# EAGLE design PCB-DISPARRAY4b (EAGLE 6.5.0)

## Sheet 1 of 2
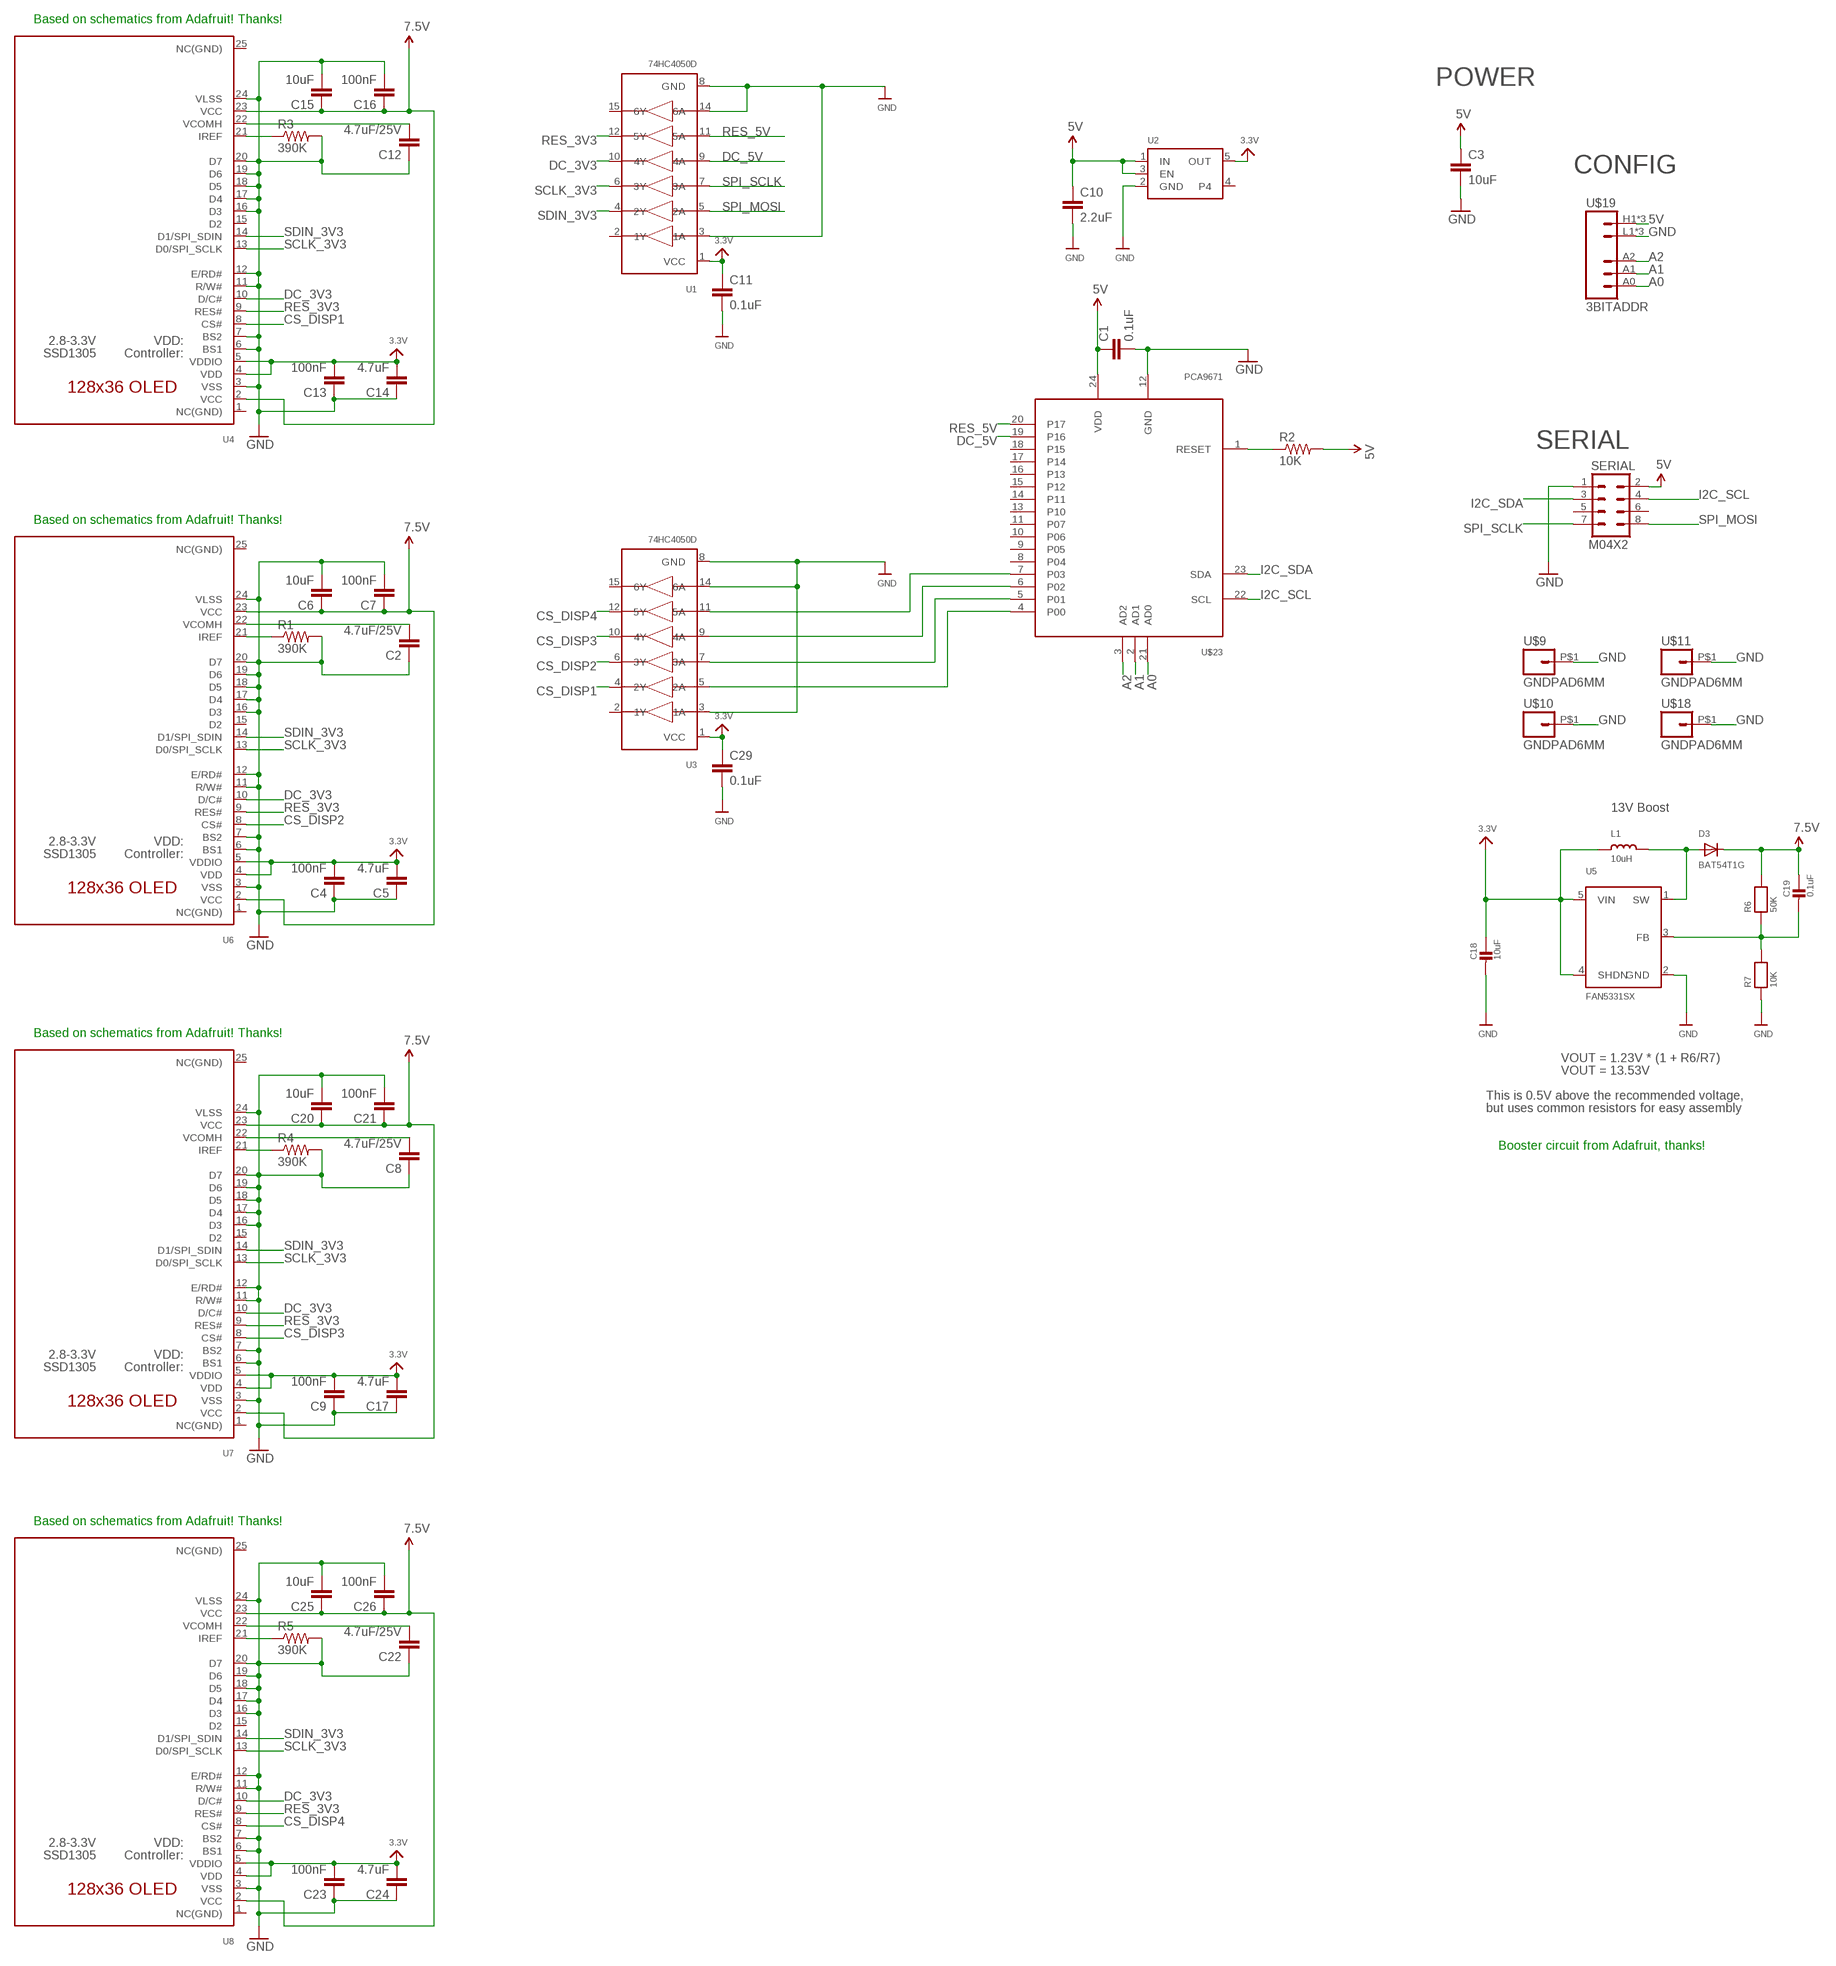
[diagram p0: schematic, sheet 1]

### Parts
C1  0.1uF  CAP0603-CAP  [0603-CAP]
C2  4.7uF/25V  CAP0805  [0805]
C3  10uF  CAP0805  [0805]
C4  100nF  CAP0603-CAP  [0603-CAP]
C5  4.7uF  CAP0603-CAP  [0603-CAP]
C6  10uF  CAP0603-CAP  [0603-CAP]
C7  100nF  CAP0603-CAP  [0603-CAP]
C8  4.7uF/25V  CAP0805  [0805]
C9  100nF  CAP0603-CAP  [0603-CAP]
C10  2.2uF  CAP0603-CAP  [0603-CAP]
C11  0.1uF  CAP0603-CAP  [0603-CAP]
C12  4.7uF/25V  CAP0805  [0805]
C13  100nF  CAP0603-CAP  [0603-CAP]
C14  4.7uF  CAP0603-CAP  [0603-CAP]
C15  10uF  CAP0603-CAP  [0603-CAP]
C16  100nF  CAP0603-CAP  [0603-CAP]
C17  4.7uF  CAP0603-CAP  [0603-CAP]
C18  10uF  CAP_CERAMIC0805  [0805]
C19  0.1uF  CAP_CERAMIC0805  [0805]
C20  10uF  CAP0603-CAP  [0603-CAP]
C21  100nF  CAP0603-CAP  [0603-CAP]
C22  4.7uF/25V  CAP0805  [0805]
C23  100nF  CAP0603-CAP  [0603-CAP]
C24  4.7uF  CAP0603-CAP  [0603-CAP]
C25  10uF  CAP0603-CAP  [0603-CAP]
C26  100nF  CAP0603-CAP  [0603-CAP]
C29  0.1uF  CAP0603-CAP  [0603-CAP]
D3  BAT54T1G  DIODESOD-123  [SOD-123]
L1  10uH  INDUCTOR  [INDUCTOR_1007]
R1  390K  RESISTOR0603-RES  [0603-RES]
R2  10K  RESISTOR0603-RES  [0603-RES]
R3  390K  RESISTOR0603-RES  [0603-RES]
R4  390K  RESISTOR0603-RES  [0603-RES]
R5  390K  RESISTOR0603-RES  [0603-RES]
R6  50K  RESISTOR0805  [0805]
R7  10K  RESISTOR0805  [0805]
SERIAL  M04X2  [2X4]
U1  74HC4050D  [SOIC16]
U2  VREG_SOT23-5  [SOT23-5]
U3  74HC4050D  [SOIC16]
U4  ER-OLED011-1  [ER-OLED011-1_WRAPAROUND]
U5  FAN5331SX  FAN5331  [SOT23-5@1]
U6  ER-OLED011-1  [ER-OLED011-1_WRAPAROUND]
U7  ER-OLED011-1  [ER-OLED011-1_WRAPAROUND]
U8  ER-OLED011-1  [ER-OLED011-1_WRAPAROUND]
U$9  GNDPAD6MM  [3.2MMPAD6MM]
U$10  GNDPAD6MM  [3.2MMPAD6MM]
U$11  GNDPAD6MM  [3.2MMPAD6MM]
U$18  GNDPAD6MM  [3.2MMPAD6MM]
U$19  3BITADDR  [3BITADDR]
U$23  PCA9671  [TSSOP24]

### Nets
3.3V: C4.2 C5.2 C9.2 C11.1 C13.2 C14.2 C17.2 C18.1 C23.2 C24.2 C29.1 L1.P$1 U1.1(VCC) U2.5(OUT) U3.1(VCC) U4.4(VDD) U4.5(VDDIO) U5.4(SHDN) U5.5(VIN) U6.4(VDD) U6.5(VDDIO) U7.4(VDD) U7.5(VDDIO) U8.4(VDD) U8.5(VDDIO)
5V [Power]: C1.1 C3.1 C10.1 R2.2 SERIAL.2 U2.1(IN) U2.3(EN) U$19.H1(VCC) U$19.H2(VCC) U$19.H3(VCC) U$23.24(VDD)
7.5V [Power]: C6.1 C7.1 C15.1 C16.1 C19.1 C20.1 C21.1 C25.1 C26.1 D3.C R6.2 U4.2(VCC) U4.23(VCC) U6.2(VCC) U6.23(VCC) U7.2(VCC) U7.23(VCC) U8.2(VCC) U8.23(VCC)
A0: U$19.A0 U$23.21(AD0)
A1: U$19.A1 U$23.2(AD1)
A2: U$19.A2 U$23.3(AD2)
CS_DISP1: U3.4(2Y) U4.8(CS#)
CS_DISP2: U3.6(3Y) U6.8(CS#)
CS_DISP3: U3.10(4Y) U7.8(CS#)
CS_DISP4: U3.12(5Y) U8.8(CS#)
DC_3V3: U1.10(4Y) U4.10(D/C#) U6.10(D/C#) U7.10(D/C#) U8.10(D/C#)
DC_5V: U1.9(4A) U$23.19(P16)
GND [Power]: C1.2 C2.1 C3.2 C4.1 C5.1 C6.2 C7.2 C8.1 C9.1 C10.2 C11.2 C12.1 C13.1 C14.1 C15.2 C16.2 C17.1 C18.2 C20.2 C21.2 C22.1 C23.1 C24.1 C25.2 C26.2 C29.2 R1.2 R3.2 R4.2 R5.2 R7.1 SERIAL.1 U1.3(1A) U1.8(GND) U1.14(6A) U2.2(GND) U3.3(1A) U3.8(GND) U3.14(6A) U4.3(VSS) U4.6(BS1) U4.7(BS2) U4.11(R/W#) U4.12(E/RD#) U4.16(D3) U4.17(D4) U4.18(D5) U4.19(D6) U4.20(D7) U4.24(VLSS) U5.2(GND) U6.3(VSS) U6.6(BS1) U6.7(BS2) U6.11(R/W#) U6.12(E/RD#) U6.16(D3) U6.17(D4) U6.18(D5) U6.19(D6) U6.20(D7) U6.24(VLSS) U7.3(VSS) U7.6(BS1) U7.7(BS2) U7.11(R/W#) U7.12(E/RD#) U7.16(D3) U7.17(D4) U7.18(D5) U7.19(D6) U7.20(D7) U7.24(VLSS) U8.3(VSS) U8.6(BS1) U8.7(BS2) U8.11(R/W#) U8.12(E/RD#) U8.16(D3) U8.17(D4) U8.18(D5) U8.19(D6) U8.20(D7) U8.24(VLSS) U$9.P$1 U$10.P$1 U$11.P$1 U$18.P$1 U$19.L1(GND) U$19.L2(GND) U$19.L3(GND) U$23.12(GND)
I2C_SCL: SERIAL.4 U$23.22(SCL)
I2C_SDA: SERIAL.3 U$23.23(SDA)
N$1: R2.1 U$23.1(RESET)
N$2: R1.1 U6.21(IREF)
N$3: C2.2 U6.22(VCOMH)
N$4: R4.1 U7.21(IREF)
N$5: R3.1 U4.21(IREF)
N$6: C8.2 U7.22(VCOMH)
N$7: R5.1 U8.21(IREF)
N$8: C22.2 U8.22(VCOMH)
N$10: C12.2 U4.22(VCOMH)
N$14: D3.A L1.P$2 U5.1(SW)
N$15: C19.2 R6.1 R7.2 U5.3(FB)
N$29: U3.5(2A) U$23.4(P00)
N$30: U3.7(3A) U$23.5(P01)
N$31: U3.9(4A) U$23.6(P02)
N$32: U3.11(5A) U$23.7(P03)
RES_3V3: U1.12(5Y) U4.9(RES#) U6.9(RES#) U7.9(RES#) U8.9(RES#)
RES_5V: U1.11(5A) U$23.20(P17)
SCLK_3V3: U1.6(3Y) U4.13(D0/SPI_SCLK) U6.13(D0/SPI_SCLK) U7.13(D0/SPI_SCLK) U8.13(D0/SPI_SCLK)
SDIN_3V3: U1.4(2Y) U4.14(D1/SPI_SDIN) U6.14(D1/SPI_SDIN) U7.14(D1/SPI_SDIN) U8.14(D1/SPI_SDIN)
SPI_MOSI: SERIAL.8 U1.5(2A)
SPI_SCLK: SERIAL.7 U1.7(3A)
Unconnected: SERIAL.5 SERIAL.6 U1.2(1Y) U1.15(6Y) U2.4 U3.2(1Y) U3.15(6Y) U4.1(NC(GND)) U4.15(D2) U4.25(NC(GND)) U6.1(NC(GND)) U6.15(D2) U6.25(NC(GND)) U7.1(NC(GND)) U7.15(D2) U7.25(NC(GND)) U8.1(NC(GND)) U8.15(D2) U8.25(NC(GND)) U$23.8(P04) U$23.9(P05) U$23.10(P06) U$23.11(P07) U$23.13(P10) U$23.14(P11) U$23.15(P12) U$23.16(P13) U$23.17(P14) U$23.18(P15)

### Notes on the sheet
- Based on schematics from Adafruit! Thanks!
- POWER
- CONFIG
- SERIAL
- Based on schematics from Adafruit! Thanks!
- 13V Boost
- Based on schematics from Adafruit! Thanks!
- VOUT = 1.23V * (1 + R6/R7)
- VOUT = 13.53V
- This is 0.5V above the recommended voltage,
- but uses common resistors for easy assembly
- Booster circuit from Adafruit, thanks!
- Based on schematics from Adafruit! Thanks!

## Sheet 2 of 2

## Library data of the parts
C1-C17 C20-C26 C29 = SparkFun:CAP: Capacitor
C18 C19 = microbuilder:CAP_CERAMIC: Ceramic Capacitors
D3 = microbuilder:DIODE: Diode
L1 = microbuilder:INDUCTOR: Inductors
R1-R5 = SparkFun:RESISTOR: Resistor
R6 R7 = microbuilder:RESISTOR: Resistors
SERIAL = SparkFun:M04X2
U1 U3 = microbuilder:74HC4050D: 6-channel level shifter 74HC4050D - 2V-6V Supply Digikey: 74HC4050D,653-ND Mouser: 771-74HC4050D-T
U2 = microbuilder:VREG_SOT23-5: SOT23-5 Fixed Voltage Regulators To better organise some of the SOT23-5 fixed voltage regulators in this library, this new part was created. Part Current Out V Out V In V Dropout Digikey Part No. ADP121 150mA 3.3V 3.4-5.5V 0.09V @ 150mA ADP121-AUJZ33R7CT-ND ADP121 150mA 3.0V 3.1-5.5V 0.09V @ 150mA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
U4 U6-U8 = SKAARHOJ:ER-OLED011-1: UG-2864HSWEG01 OLED display Both 1.3" and 0.96" models share the same FPC tab footprint, only the screen dimensions vary.
U5 = microbuilder:FAN5331: FAN5331 - LED/OLED 20V Boost Converter Digikey: FAN5331SXCT-ND
U$9-U$11 U$18 = SKAARHOJ:GNDPAD
U$19 = SKAARHOJ:3BITADDR
U$23 = SKAARHOJ:PCA9671

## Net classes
0 default: width 0.203 mm, drill 0.406 mm, clearance 0.152 mm
1 Power: width 0.203 mm, drill 0.61 mm, clearance 0.152 mm
2 RELAY LINES: width 0.305 mm, drill 0.406 mm, clearance 0.254 mm
3 INput lines: width 0.203 mm, drill 0.406 mm, clearance 0.254 mm

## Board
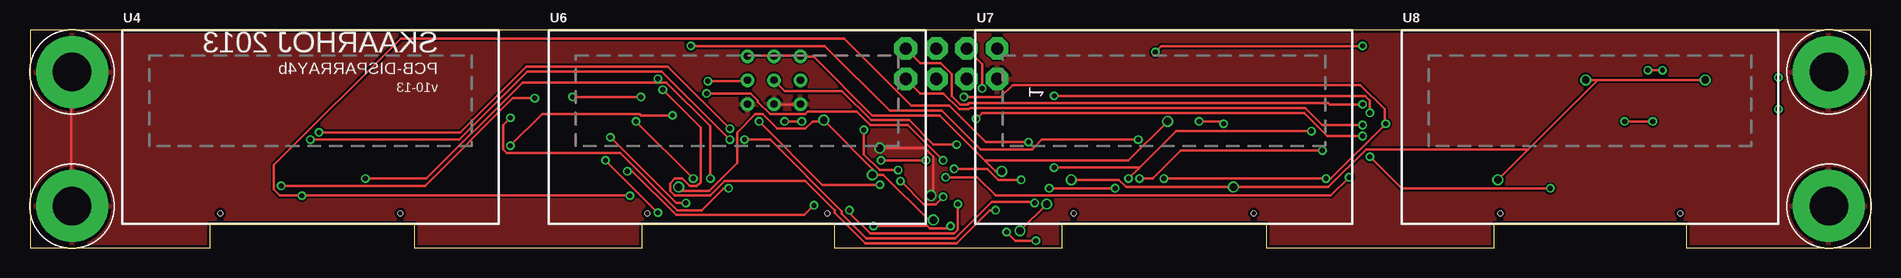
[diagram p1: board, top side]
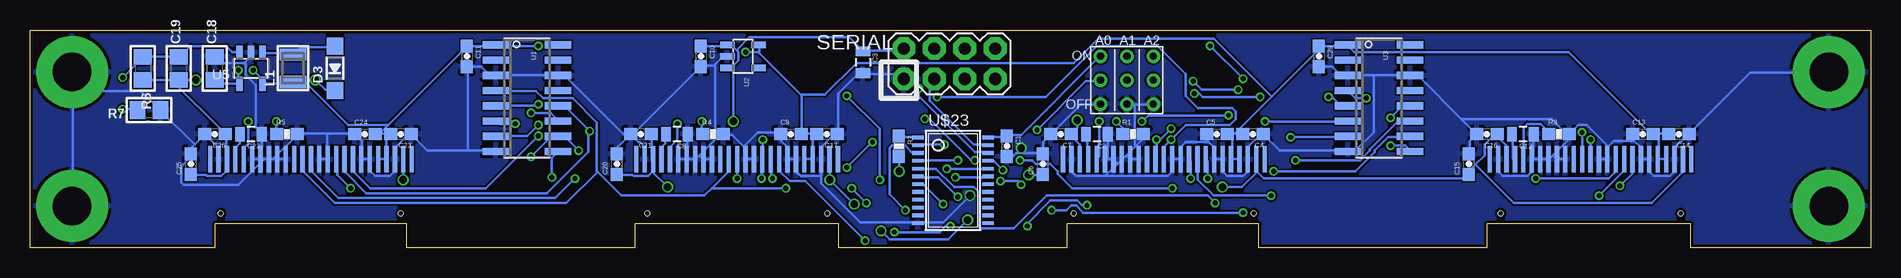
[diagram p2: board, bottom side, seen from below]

Size 153.42 x 18.2 mm. Coordinates in mm from the lower left corner, seen from the top.
Outline: 153.42,0 153.42,18.2 0,18.2 0,0 15,0 15,2 32,2 32,0 51,0 51,2 67,2 67,0 86,0 86,2 103,2 103,0 122,0 122,2 138,2 138,0 153.42,0
Copper layers (1*16): Top 0.035mm / dielectric 1.5mm / Bottom 0.035mm
Design rules "Fusion_eagle_rule_v1.1": minimum track width 6mil, minimum drill 12mil, track to track 6mil, track to pad 6mil, pad to pad 6mil, via to via 6mil, smd to smd 0mil, copper to edge 10mil, drill to drill 10mil, minimum pad ring 10mil, minimum via ring 6mil, stop-mask expansion 2mil, vias tented up to drill 100mil, thermal gap 10mil

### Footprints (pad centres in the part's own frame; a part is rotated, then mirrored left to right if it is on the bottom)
0603-CAP = smd 1.1 x 1: 1 -0.85,0; 2 0.85,0
0805 = smd 0.8 x 1.2: 1 -0.9,0; 2 0.9,0
0805' = smd 1.3 x 1.5: 1 -0.95,0; 2 0.95,0
SOD-123 = smd 1.4 x 1.4: A 1.85,0; C -1.85,0
INDUCTOR_1007 = smd 1.016 x 2.2: P$1 -1.127,0; P$2 1.127,0
0603-RES = smd 1.1 x 1: 1 -0.85,0; 2 0.85,0
2X4 = drill 1.016 pad 1.88 octagon: 1 -3.81,-1.27; 2 -3.81,1.27; 3 -1.27,-1.27; 4 -1.27,1.27; 5 1.27,-1.27; 6 1.27,1.27; 7 3.81,-1.27; 8 3.81,1.27
SOIC16 = smd 0.6 x 2.2: 1 -4.445,-2.6; 2 -3.175,-2.6; 3 -1.905,-2.6; 4 -0.635,-2.6; 5 0.635,-2.6; 6 1.905,-2.6; 7 3.175,-2.6; 8 4.445,-2.6; 9 4.445,2.6; 10 3.175,2.6; 11 1.905,2.6; 12 0.635,2.6; 13 -0.635,2.6; 14 -1.905,2.6; 15 -3.175,2.6; 16 -4.445,2.6
SOT23-5 = smd 0.55 x 1.2: 1 -0.95,-1.3; 2 0,-1.3; 3 0.95,-1.3; 4 0.95,1.3; 5 -0.95,1.3
ER-OLED011-1_WRAPAROUND = smd 0.35 x 2.2 bottom: 1 -8.4,-2.7; 2 -7.7,-2.7; 3 -7,-2.7; 4 -6.3,-2.7; 5 -5.6,-2.7; 6 -4.9,-2.7; 7 -4.2,-2.7; 8 -3.5,-2.7; 9 -2.8,-2.7; 10 -2.1,-2.7; 11 -1.4,-2.7; 12 -0.7,-2.7; 13 0,-2.7; 14 0.7,-2.7; 15 1.4,-2.7; 16 2.1,-2.7; 17 2.8,-2.7; 18 3.5,-2.7; 19 4.2,-2.7; 20 4.9,-2.7; 21 5.6,-2.7; 22 6.3,-2.7; 23 7,-2.7; 24 7.7,-2.7; 25 8.4,-2.7 | hole 0.4: -7.5,-7.2; 7.5,-7.2
SOT23-5@1 = smd 0.55 x 1.2: 1 -0.95,-1.3; 2 0,-1.3; 3 0.95,-1.3; 4 0.95,1.3; 5 -0.95,1.3
3.2MMPAD6MM = drill 3.2 pad 6: P$1 0,0
3BITADDR = drill 0.6: A0 -2.2,0; A1 0,0; A2 2.2,0; H1 -2.2,2; H2 0,2; H3 2.2,2; L1 -2.2,-2; L2 0,-2; L3 2.2,-2
TSSOP24 = smd 0.305 x 0.991: 1 -4.225,-2.918; 2 -3.575,-2.918; 3 -2.925,-2.918; 4 -2.275,-2.918; 5 -1.625,-2.918; 6 -0.975,-2.918; 7 -0.325,-2.918; 8 0.325,-2.918; 9 0.975,-2.918; 10 1.625,-2.918; 11 2.275,-2.918; 12 2.925,-2.918; 13 2.925,2.918; 14 2.275,2.918; 15 1.625,2.918; 16 0.975,2.918; 17 0.325,2.918; 18 -0.325,2.918; 19 -0.975,2.918; 20 -1.625,2.918; 21 -2.275,2.918; 22 -2.925,2.918; 23 -3.575,2.918; 24 -4.225,2.918

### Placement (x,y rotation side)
C1  72,8.5 270 bottom
C2  64.5,9.5 180 bottom
C3  84,15.5 270 bottom
C4  51.5,9.5 180 bottom
C5  54.5,9.5 0 bottom
C6  69,7 90 bottom
C7  67.5,9.5 180 bottom
C8  99.5,9.5 180 bottom
C9  90,9.5 0 bottom
C10  97.5,16 270 bottom
C11  117,16 270 bottom
C12  29,9.5 180 bottom
C13  19,9.5 0 bottom
C14  16,9.5 180 bottom
C15  33.5,7 90 bottom
C16  32,9.5 180 bottom
C17  87,9.5 180 bottom
C18  10uF  [0805']  138,15 90 bottom
C19  0.1uF  [0805']  141,15 90 bottom
C20  104.5,7 90 bottom
C21  102.5,9.5 180 bottom
C22  135,9.5 180 bottom
C23  122.5,9.5 180 bottom
C24  125.5,9.5 0 bottom
C25  140,7 90 bottom
C26  138,9.5 180 bottom
C29  46,16 270 bottom
D3  128,15 90 bottom
L1  131.5,15 90 bottom
R1  61.5,9.5 0 bottom
R2  81,8.5 270 bottom
R3  26,9.5 0 bottom
R4  96.5,9.5 0 bottom
R5  132,9.5 0 bottom
R6  50K  [0805']  144,15 270 bottom
R7  10K  [0805']  143.5,11.5 180 bottom
SERIAL  76.79,15.38 0 bottom
U1  112,12.5 270 bottom
U2  94,16 270 bottom
U3  41,12.5 270 bottom
U4  23.37,10.1 0 top
U5  135,15 180 bottom
U6  58.93,10.1 0 top
U7  94.49,10.1 0 top
U8  130,10.1 0 top
U$9  149.92,3.5 0 top
U$10  3.5,3.5 0 top
U$11  149.92,14.7 0 top
U$18  3.5,14.7 0 top
U$19  62,14 0 bottom
U$23  76.5,5 270 bottom

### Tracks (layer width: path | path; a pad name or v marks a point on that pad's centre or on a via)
3.3V  (via drill 0.41)
  Top 0.203: v134.82,14.83 v136.04,14.83 | v111.05,16.87 94.28,16.87 v93.78,16.36
  Bottom 0.203: C18.1 137.97,14.02 137.67,13.72 136.04,13.72 U5.4 136.04,13.82 v136.04,14.83 | 133.71,13.72 131.67,13.72 131.57,13.82 L1.P$1 131.47,13.82 130.45,13.82 126.9,10.26 123.65,10.26 123.6,10.21 | 133.71,13.72 134.01,13.72 U5.5 | 133.71,13.72 v134.82,14.83 | 124.26,9.55 124.56,9.55 C24.2 124.26,9.55 | 124.26,9.55 123.75,9.55 | 123.75,9.55 123.44,9.55 C23.2 123.75,9.55 | 123.75,9.55 123.75,7.42 U8.4 123.85,7.42 124.36,7.42 U8.5 | 124.26,9.55 123.6,10.21 | 123.6,10.21 117.04,16.76 C11.1 116.94,16.87 114.61,16.87 U1.1 114.5,16.87 v111.05,16.87 | U7.5 88.8,7.42 88.19,7.42 U7.4 88.19,7.52 88.19,9.55 | 88.19,9.55 89.1,9.55 C9.2 89.1,9.65 89.1,12.7 89.15,12.75 | 88.19,9.55 87.88,9.55 C17.2 88.19,9.55 | 92.66,16.36 92.66,16.26 89.15,12.75 | 92.66,16.36 92.66,16.87 U2.5 | 17.68,9.55 18.09,9.55 C13.2 | 17.68,9.55 16.87,9.55 C14.2 | 17.68,7.42 17.68,9.55 | 17.68,9.55 C13.2 | 17.68,7.42 U4.5 | 17.68,7.42 17.07,7.42 U4.4 | 53.24,9.55 53.65,9.55 C5.2 53.24,9.55 | 53.24,9.55 53.03,9.55 | 53.03,9.55 52.43,9.55 C4.2 | 53.24,7.42 53.24,9.55 | 53.24,7.42 U6.5 | 53.24,7.42 52.63,7.42 U6.4 | 53.03,9.55 49.94,12.65 | 49.94,12.65 46.02,16.56 46.02,16.76 C29.1 45.92,16.87 43.69,16.87 U3.1 43.59,16.87 43.08,16.36 25.2,16.36 18.39,9.55 18.19,9.55 C13.2 | 49.94,12.65 54.76,17.48 64.41,17.48 66.45,15.44 84.53,15.44 87.17,12.8 89.1,12.8 89.15,12.75 | 92.66,16.36 v93.78,16.36
5V  (via drill 0.61)
  Top 0.203: U$19.H3 59.84,16.05 61.98,16.05 U$19.H2 62.08,16.05 64.11,16.05 U$19.H1 64.21,15.95 65.33,15.95 70.21,11.07 75.79,11.07 79.6,7.26 | v80.97,6.4 80.47,6.4 79.6,7.26 | v94.79,10.57 91.54,7.32 79.65,7.32 79.6,7.26
  Bottom 0.203: C10.1 97.43,16.87 95.3,16.87 U2.1 95.2,16.87 94.89,16.87 94.54,16.51 | 94.54,16.51 94.39,16.36 94.39,15.65 94.89,15.14 95.2,15.14 U2.3 94.79,15.14 v94.79,10.57 | SERIAL.2 80.67,16.56 80.77,16.46 83.92,16.46 C3.1 84.02,16.46 85.14,17.58 93.47,17.58 94.54,16.51 | U$23.24 73.56,9.25 72.14,9.25 72.03,9.35 C1.1 71.93,9.45 70.81,9.45 64.21,16.05 U$19.H1 | v80.97,6.4 80.97,7.62 R2.2
7.5V  (via drill 0.61)
  Top 0.203: v54.05,5.08 54.36,4.78 56.59,4.78 58.93,7.11 58.93,9.65 60.45,11.18 61.06,11.18 62.28,9.96 64.62,9.96 65.23,10.57 66.14,10.57 v66.14,10.67 70.21,6.6 v70.21,6.1 71.12,6.1 74.88,2.34 v75.29,2.34 | v86.77,5.69 90.73,5.69 91.34,5.08 v100.28,5.08 108.2,5.08 111.35,8.23 124.77,8.23 124.82,8.18 | v139.6,14.02 130.66,14.02 | 130.66,14.02 v129.64,14.02 | 130.66,14.02 124.82,8.18 | 124.82,8.18 v122.33,5.69 | v84.73,3.66 v82.5,1.42
  Bottom 0.203: 65.94,7.42 U6.23 65.94,7.52 65.94,8.64 66.75,9.45 C7.1 66.65,9.55 66.14,10.06 v66.14,10.67 | v70.21,6.1 69.09,6.1 C6.1 | 51.21,7.42 U6.2 51.21,7.32 51.21,6.4 51.16,6.35 | 30.38,7.42 U4.23 30.38,7.52 30.38,8.53 31.19,9.35 C16.1 31.19,9.45 31.39,9.45 32.21,8.64 32.21,7.72 32.97,6.96 | 32.97,6.96 33.43,6.5 33.43,6.2 C15.1 33.53,6.1 33.83,5.79 50.6,5.79 51.16,6.35 | 32.97,6.96 29.77,3.76 18.29,3.76 15.75,6.3 15.75,7.32 U4.2 | v54.05,5.08 52.43,5.08 51.16,6.35 | 86.77,7.42 U7.2 86.77,7.32 v86.77,5.69 v84.73,3.66 | 101.55,6.35 101.5,6.4 101.5,7.32 U7.23 | 101.55,6.35 101.91,5.99 103.12,5.99 103.23,6.1 104.44,6.1 C20.1 | C21.1 101.6,9.45 101.6,7.32 U7.23 | 101.55,6.35 v100.28,5.08 | 101.5,7.42 U7.23 | C25.1 139.9,6.1 138.79,6.1 138.68,5.99 137.47,5.99 137.06,6.4 137.06,7.32 U8.23 137.06,7.42 137.06,9.45 C26.1 137.16,9.55 141.63,14.02 | 122.33,7.42 U8.2 122.33,7.32 v122.33,5.69 | v129.64,14.02 128.83,13.21 128.02,13.21 D3.C | v139.6,14.02 140.92,14.02 C19.1 | 141.63,14.02 141.02,14.02 C19.1 | 141.63,14.02 143.97,14.02 R6.2 | 141.63,14.02 C19.1 | v75.29,2.34 76.91,0.71 81.79,0.71 v82.5,1.42
A0  (via drill 0.41)
  Top 0.203: v72.34,6.5 70.81,6.5 69.49,7.82 v69.49,9.86
  Bottom 0.203: v72.34,6.5 73.05,7.21 73.56,7.21 U$23.21 | v69.49,9.86 65.43,13.92 64.21,13.92 U$19.A0
A1  (via drill 0.41)
  Top 0.203: v77.22,8.64 75.29,8.64 73.25,10.67 70.1,10.67 67.67,13.11 62.89,13.11 62.08,13.92 U$19.A1
  Bottom 0.203: v77.22,8.64 79.35,8.64 U$23.2
A2  (via drill 0.41)
  Top 0.203: v80.47,3.15 79.96,3.15 77.22,0.41 69.6,0.41 67.06,2.95 67.06,3.15 64.62,5.59 57.91,5.59 56.69,4.37 53.75,4.37 53.34,4.78 53.34,5.38 53.75,5.79 54.36,5.79 54.97,5.18 55.58,5.18 55.88,5.49 55.88,10.06 v52.73,13.21 | v56.49,13.92 59.74,13.92 U$19.A2
  Bottom 0.203: v80.47,3.15 81.79,4.47 81.79,8.33 81.58,8.53 80.47,8.53 79.96,8.03 79.45,8.03 U$23.3 | v52.73,13.21 55.78,13.21 v56.49,13.92
CS_DISP1  (via drill 0.41)
  Top 0.203: v20.93,5.18 32.92,5.18 40.23,12.5 v42.06,12.5
  Bottom 0.203: v20.93,5.18 19.91,6.2 19.91,7.32 U4.8 | v42.06,12.5 42.98,12.5 43.59,13.11 U3.4
CS_DISP2  (via drill 0.41)
  Top 0.203: v55.27,5.79 v50.49,10.57
  Bottom 0.203: v50.49,10.57 43.69,10.57 U3.6 | v55.27,5.79 55.27,7.21 55.37,7.32 U6.8
CS_DISP3  (via drill 0.41)
  Top 0.203: v49.78,6.4 50.19,6.4 53.85,2.74 64.52,2.74 v65.33,3.56 | v70.31,1.83 74.78,1.83 74.98,1.63 76.5,1.63 v76.71,1.83 | v81.38,1.32 82.09,0.61 v83.82,0.61
  Bottom 0.203: v49.78,6.4 42.98,6.4 41.35,8.03 41.35,8.13 40.23,9.25 38.41,9.25 U3.10 | v65.33,3.56 65.73,3.56 66.14,3.96 68.38,3.96 70.31,2.03 v70.31,1.83 | v76.71,1.83 77.11,1.83 77.62,1.32 v81.38,1.32 | v83.82,0.61 88.8,5.59 90.12,5.59 90.93,6.4 90.93,7.32 U7.8
CS_DISP4  (via drill 0.41)
  Top 0.203: v111.05,9.35 108.1,9.35 106.17,11.28 79.35,11.28 v78.84,10.77 | v70.92,7.32 v74.68,7.32 | v58.22,4.98 57.81,4.98 55.98,3.15 53.95,3.15 49.17,7.92 39.73,7.92 39.42,8.23 39.42,10.26 v40.03,10.87
  Bottom 0.203: v111.05,9.35 115.42,4.98 125.07,4.98 126.49,6.4 126.49,7.32 U8.8 | v78.84,10.77 78.44,10.77 74.98,7.32 v74.68,7.32 | v70.92,7.32 69.9,7.32 69.6,7.01 68.38,7.01 67.77,6.4 67.77,6.2 66.55,4.98 v58.22,4.98 | v40.03,10.87 39.12,11.79 38.41,11.79 U3.12
DC_3V3  (via drill 0.41)
  Top 0.203: v92.46,5.79 93.57,5.79 95.91,8.13 v107.7,8.13 | v126.69,4.98 114.3,4.98 v111.66,7.62 | v27.94,5.79 33.02,5.79 41.05,13.82 52.32,13.82 | 52.32,13.82 53.03,13.82 56.69,10.16 v56.69,5.79 | v92.35,9.04 84.33,9.04 83.52,8.23 79.25,8.23 76,11.48 71.63,11.48 66.24,16.87 v55.07,16.87 | 52.32,13.82 v52.32,14.12
  Bottom 0.203: v92.46,5.79 92.46,7.32 U7.10 92.35,7.42 v92.35,9.04 | v107.7,8.13 108.81,9.25 109.32,9.25 U1.10 109.42,9.25 110.03,9.25 v111.66,7.62 | v126.69,4.98 127.81,6.1 127.81,7.32 U8.10 | v27.94,5.79 21.84,5.79 21.34,6.3 21.34,7.32 U4.10 | v56.69,5.79 56.69,7.21 56.79,7.32 U6.10 | v52.32,14.12 v55.07,16.87
DC_5V  (via drill 0.41)
  Top 0.203: v76.3,5.89 78.94,5.89 80.47,4.37 108.41,4.37 v109.93,5.89
  Bottom 0.203: v76.3,5.89 73.66,5.89 U$23.19 | v109.93,5.89 109.93,7.52 109.42,8.03 U1.9
GND  (via drill 0.61)
  Top 0.203: U$10.P$1 3.45,3.56 3.45,14.63 U$18.P$1 | U$19.L1 64.11,11.99 62.08,11.99 U$19.L2 | v70.81,8.33 74.57,8.33 75.29,7.62 75.29,4.57 v75.08,4.37
  Bottom 0.203: 70.81,7.92 69.09,7.92 C6.2 68.99,7.92 68.99,8.84 68.38,9.45 C7.2 68.28,9.55 65.84,11.99 U$19.L1 | 70.81,7.92 71.22,7.92 71.42,7.72 71.93,7.72 C1.2 | 61.37,11.99 61.98,11.99 U$19.L2 | 61.37,11.99 59.84,11.99 U$19.L3 | 55.22,8.89 54.76,8.43 54.76,7.42 U6.7 54.66,7.42 54.05,7.42 U6.6 53.95,7.32 53.95,6.3 53.65,5.99 52.32,5.99 52.02,6.3 52.02,7.32 U6.3 51.92,7.42 51.92,8.43 50.9,9.45 50.7,9.45 C4.1 50.6,9.45 49.28,8.13 43.69,8.13 U3.8 43.59,8.13 42.98,8.13 41.45,9.65 41.45,14.43 | 55.22,8.89 55.27,8.94 55.27,9.45 C5.1 | 55.22,8.89 55.27,8.84 57.1,8.84 57.61,8.33 57.61,7.52 U6.11 57.61,7.42 58.22,7.42 U6.12 58.32,7.32 58.32,6.3 58.62,5.99 63.7,5.99 63.75,6.04 | C2.1 63.6,9.45 63.6,7.62 63.8,7.42 U6.20 63.7,7.42 63.2,7.42 U6.19 63.09,7.32 62.79,7.01 | U6.16 61.06,7.42 61.67,7.42 U6.17 61.77,7.42 62.08,7.72 | 62.08,7.72 62.38,7.42 U6.18 62.48,7.32 62.79,7.01 | 62.08,7.72 61.32,8.48 | 61.32,8.48 60.66,9.14 60.66,9.45 R1.2 | 62.79,7.01 63.75,6.04 | 63.75,6.04 63.8,5.99 66.24,5.99 66.55,6.3 66.55,7.32 U6.24 | 61.37,11.99 61.37,8.53 61.32,8.48 | U4.16 25.5,7.42 26.11,7.42 U4.17 26.21,7.42 26.52,7.72 | 26.52,7.72 26.82,7.42 U4.18 26.92,7.42 27.53,7.42 U4.19 27.64,7.42 28.14,7.42 U4.20 | 26.52,7.72 25.2,9.04 25.2,9.45 R3.2 | C12.1 28.14,9.45 28.14,7.52 28.25,7.42 U4.20 | U4.24 30.99,7.32 30.99,6.3 30.68,5.99 28.65,5.99 28.35,6.3 28.35,7.32 U4.20 | U4.12 22.66,7.42 22.05,7.42 U4.11 22.05,7.52 22.05,8.33 21.89,8.48 | 19.76,8.99 19.2,8.43 19.2,7.42 U4.7 19.1,7.42 18.49,7.42 U4.6 18.39,7.32 18.39,6.3 18.09,5.99 16.76,5.99 16.46,6.3 16.46,7.32 U4.3 16.36,7.42 16.36,8.43 15.95,8.84 15.85,8.84 15.24,9.45 C14.1 15.14,9.55 10.06,14.63 3.56,14.63 U$18.P$1
  Bottom 0.203: 19.76,8.99 19.81,9.04 19.81,9.45 C13.1 | 21.89,8.48 21.44,8.94 19.81,8.94 19.76,8.99 | 21.89,8.48 23.67,10.26 24.38,10.26 25.09,9.55 R3.2 | C29.2 45.92,15.14 44.91,15.14 44.2,14.43 43.69,14.43 U3.3 43.59,14.43 41.45,14.43 | C15.2 33.43,7.92 33.43,8.94 32.92,9.45 C16.2 32.92,9.55 34.09,10.72 | 34.09,10.72 37.69,14.33 38.3,14.33 U3.14 38.41,14.43 41.45,14.43 | R3.2 25.3,9.45 26.62,10.77 34.04,10.77 34.09,10.72 | 139.7,8.64 138.89,9.45 C26.2 138.79,9.45 137.77,8.43 137.77,7.42 U8.24 | 139.7,8.64 139.9,8.43 139.9,7.92 C25.2 140,7.82 140,7.62 140.82,6.81 140.82,5.49 140.61,5.28 136.04,5.28 133.91,7.42 | 139.7,8.64 142.54,11.48 R7.1 142.65,11.58 144.17,13.11 148.34,13.11 149.86,14.63 U$11.P$1 149.86,14.53 149.86,3.56 U$9.P$1 | U8.12 129.24,7.42 128.63,7.42 U8.11 128.63,7.52 128.63,9.55 | 128.63,9.55 131.06,9.55 R5.2 131.17,9.45 133.2,7.42 | 128.63,9.55 126.39,9.55 C24.1 126.29,9.45 125.78,8.94 125.78,7.52 U8.7 125.78,7.42 125.17,7.42 U8.6 125.07,7.32 125.07,6.4 124.66,5.99 123.44,5.99 123.04,6.4 123.04,7.32 U8.3 122.94,7.42 122.94,8.43 121.92,9.45 121.72,9.45 C23.1 121.61,9.45 120.29,8.13 116.94,8.13 | 135.48,15.49 135.53,15.44 137.57,15.44 137.97,15.85 C18.2 | 135.48,15.49 135.03,15.95 135.03,16.26 U5.2 | U8.16 132.18,7.42 132.79,7.42 U8.17 132.89,7.42 133.2,7.42 | 134.11,7.42 134.11,9.45 C22.1 134.11,9.55 134.62,10.06 134.62,13.61 135.43,14.43 135.43,15.44 135.48,15.49 | 134.11,7.42 U8.19 134.21,7.42 134.82,7.42 U8.20 | 133.91,7.42 133.5,7.42 U8.18 133.4,7.42 133.2,7.42 | 133.91,7.42 134.11,7.42 | 116.94,8.13 114.61,8.13 U1.8 | 116.94,8.13 116.94,15.04 C11.2 116.94,15.14 115.82,15.14 115.11,14.43 114.61,14.43 U1.3 114.5,14.43 109.42,14.43 U1.14 109.32,14.33 108.81,14.33 103.73,9.25 C21.2
  Bottom 0.203: C20.2 104.44,7.92 104.44,8.43 103.43,9.45 C21.2 | C21.2 103.33,9.45 102.72,8.84 102.62,8.84 102.21,8.43 102.21,7.42 U7.24 | C8.1 98.65,9.45 98.65,7.42 U7.19 | U7.20 99.36,7.42 98.75,7.42 U7.19 | U7.16 96.62,7.42 97.23,7.42 U7.17 97.33,7.42 97.64,7.72 | U7.11 93.17,7.42 93.78,7.42 U7.12 93.78,7.52 93.78,8.33 93.93,8.48 | 96.37,15.29 95.71,15.95 95.3,15.95 U2.2 | 96.37,15.29 96.42,15.24 97.43,15.24 C10.2 97.54,15.14 103.23,9.45 C21.2 | 97.64,7.72 97.94,7.42 U7.18 98.04,7.42 98.55,7.42 U7.19 | 97.64,7.72 96.27,9.09 | 96.27,9.09 95.91,9.45 95.71,9.45 R4.2 95.61,9.45 94.89,9.45 93.93,8.48 | 96.37,15.29 96.32,15.24 96.32,9.14 96.27,9.09 | SERIAL.1 80.67,14.12 81.08,14.53 83.92,14.53 C3.2 84.02,14.53 84.43,14.53 86.06,12.9 86.06,9.55 C17.1 86.16,9.45 86.46,9.45 87.48,8.43 87.48,7.42 U7.3 87.48,7.32 87.48,5.99 | 87.48,5.99 87.48,5.38 84.23,2.13 79.45,2.13 U$23.12 79.35,2.13 77.32,2.13 v75.08,4.37 | 87.48,5.99 89.2,5.99 89.51,6.3 89.51,7.32 U7.6 89.61,7.42 90.22,7.42 U7.7 90.32,7.42 90.32,8.43 90.83,8.94 90.83,9.45 C9.1 90.93,9.55 91.03,9.65 92.76,9.65 93.93,8.48 | v70.81,8.33 70.81,7.92
  pour Top: 0,0 153,0 153,18 0,18
  pour Bottom: 0,0 153,0 153,18 0,18
I2C_SCL  (via drill 0.41)
  Top 0.203: v79.35,13.31 79.35,15.34 78.13,16.56 SERIAL.4
  Bottom 0.203: v79.35,13.31 79.35,12.7 74.68,8.03 73.66,8.03 U$23.22
I2C_SDA
  Bottom 0.203: U$23.23 73.66,8.64 74.78,8.64 78.44,12.29 78.44,13.72 78.13,14.02 SERIAL.3
N$1
  Bottom 0.203: U$23.1 79.45,9.25 80.87,9.25 80.97,9.35 R2.1
N$2  (via drill 0.41)
  Top 0.203: v64.31,10.57 v62.89,10.57
  Bottom 0.203: v62.89,10.57 62.38,10.06 62.38,9.55 R1.1 | v64.31,10.57 64.31,7.62 64.52,7.42 U6.21
N$3
  Bottom 0.203: C2.2 65.33,9.45 65.33,7.42 U6.22
N$4  (via drill 0.41)
  Top 0.203: v97.43,10.57 99.26,10.57 v99.47,10.36
  Bottom 0.203: v97.43,10.57 97.43,9.55 R4.1 | v99.47,10.36 99.47,9.04 100.08,8.43 100.08,7.42 U7.21
N$5
  Bottom 0.203: R3.1 26.92,9.55 26.92,9.75 27.53,10.36 28.65,10.36 28.96,10.06 28.96,7.42 U4.21
N$6
  Bottom 0.203: C8.2 100.48,9.45 100.48,8.74 100.79,8.43 100.79,7.42 U7.22
N$7  (via drill 0.41)
  Top 0.203: v135.23,10.57 v132.89,10.57
  Bottom 0.203: v132.89,10.57 132.89,9.55 R5.1 | v135.23,10.57 135.23,8.74 135.53,8.43 135.53,7.42 U8.21
N$8
  Bottom 0.203: C22.2 135.94,9.45 135.94,8.74 136.25,8.43 136.25,7.42 U8.22
N$10
  Bottom 0.203: C12.2 29.87,9.45 29.87,7.52 29.77,7.42 U4.22
N$14
  Bottom 0.203: U5.1 134.01,16.26 131.67,16.26 131.57,16.15 L1.P$2 131.47,16.15 130.86,16.76 128.02,16.76 D3.A
N$15  (via drill 0.41)
  Top 0.203: v145.69,14.22 v145.69,11.58
  Bottom 0.203: U5.3 136.04,16.36 136.55,16.36 137.06,16.87 140,16.87 140.92,15.95 C19.2 141.02,15.95 143.97,15.95 R6.1 144.07,15.85 v145.69,14.22 | v145.69,11.58 144.47,11.58 R7.2
N$29  (via drill 0.41)
  Top 0.203: v76.1,7.32 73.15,10.26 70,10.26 68.89,11.38 64.82,11.38 64.62,11.18 61.67,11.18 60.66,12.19 60.66,12.29 60.05,12.9 v56.39,12.9 | v45.21,12.6 v50.9,12.6
  Bottom 0.203: v76.1,7.32 79.35,7.32 U$23.4 | v56.39,12.9 55.98,12.9 55.68,12.6 v50.9,12.6 | v45.21,12.6 44.91,12.6 44.2,11.89 43.69,11.89 U3.5
N$30  (via drill 0.41)
  Top 0.203: v54.66,3.76 53.85,3.76 v48.36,9.25
  Bottom 0.203: v54.66,3.76 55.27,4.37 68.68,4.37 71.42,1.63 74.17,1.63 74.37,1.83 74.37,4.67 74.78,5.08 76.4,5.08 77.93,6.6 79.35,6.6 U$23.5 | v48.36,9.25 43.69,9.25 U3.7
N$31  (via drill 0.41)
  Top 0.203: v76.1,4.27 75.49,3.66 74.47,3.66 v72.54,5.59 | v70.81,5.28 66.04,5.28 v60.76,10.57 | v53.54,11.07 50.9,11.07 50.8,11.18 42.67,11.18 v40.03,8.53
  Bottom 0.203: v76.1,4.27 77.72,5.89 79.35,5.89 U$23.6 | v72.54,5.59 71.12,5.59 v70.81,5.28 | v60.76,10.57 60.25,11.07 v53.54,11.07 | v40.03,8.53 38.81,8.53 38.41,8.13 U3.9
N$32  (via drill 0.41)
  Top 0.203: v77.32,3.66 77.32,1.52 77.01,1.22 70,1.22 68.28,2.95 v68.28,3.15 | v47.95,7.32 v52.32,2.95
  Bottom 0.203: v77.32,3.66 78.94,5.28 79.35,5.28 U$23.7 | v68.28,3.15 67.06,3.15 66.65,3.56 66.24,3.56 65.63,2.95 v52.32,2.95 | v47.95,7.32 42.57,7.32 41.76,8.13 41.76,8.23 39.42,10.57 38.41,10.57 U3.11
RES_3V3  (via drill 0.41)
  Top 0.203: v49.99,4.37 v22.66,4.37 20.83,4.37 20.32,4.88 20.32,6.91 30.89,17.48 67.87,17.48 73.46,11.89 76.61,11.89 79.65,8.84 v83.21,8.84 | 92.41,6.66 95.5,9.75 v106.78,9.75 | 92.41,6.66 v91.54,5.79 | v85.34,6.71 92.35,6.71 92.41,6.66
  Bottom 0.203: v22.66,4.37 20.62,6.4 20.62,7.32 U4.9 | v49.99,4.37 54.76,4.37 56.08,5.69 56.08,7.32 U6.9 | v91.54,5.79 91.64,5.89 91.64,7.32 U7.9 | U1.12 109.32,11.79 108.81,11.79 v106.78,9.75 106.88,9.75 106.88,8.03 110.34,4.57 125.37,4.57 127.1,6.3 127.1,7.32 U8.9 | v85.34,6.71 v83.21,8.84
RES_5V  (via drill 0.41)
  Top 0.203: v77.01,6.6 79.76,6.6 80.67,5.69 v82.6,5.69 | v85.34,12.7 111.25,12.7 111.66,12.29 v111.66,11.28
  Bottom 0.203: v77.01,6.6 73.66,6.6 U$23.20 | v82.6,5.69 82.6,9.96 v85.34,12.7 | v111.66,11.28 110.03,11.28 109.42,10.67 U1.11
SCLK_3V3  (via drill 0.41)
  Top 0.203: v94.49,5.79 v108,5.79 108.41,5.79 v112.98,10.36 112.88,10.36 112.88,11.58 110.85,13.61 81.89,13.61 80.87,12.6 v77.83,12.6 | v23.37,9.04 35.76,9.04 41.45,14.73 52.63,14.73 v58.32,9.04
  Bottom 0.203: v94.49,5.79 U7.13 | v112.98,10.36 114.3,10.36 114.5,10.57 U1.6 | v108,5.79 109.63,4.17 127.71,4.17 129.95,6.4 129.95,7.32 U8.13 | v23.37,9.04 U4.13 | U6.13 58.93,8.43 v58.32,9.04 57.1,10.26 53.44,10.26 52.93,10.77 52.93,11.38 53.24,11.68 56.08,11.68 57.1,12.7 57.1,14.53 59.44,16.87 64.52,16.87 68.78,12.6 v77.83,12.6
SDIN_3V3  (via drill 0.41)
  Top 0.203: v24.08,9.65 35.87,9.65 41.35,15.14 53.14,15.14 v58.32,9.96 | v59.54,9.04 61.67,9.04 67.67,3.05 67.67,2.85 69.7,0.81 77.11,0.81 80.16,3.86 83.62,3.86 v83.72,3.76 | v90.42,4.98 v84.94,4.98
  Bottom 0.203: v24.08,9.65 24.08,7.42 U4.14 | 59.38,8.89 59.54,8.74 59.54,7.42 U6.14 | 59.38,8.89 v58.32,9.96 | 96.57,5.03 97.23,4.37 104.14,4.37 106.12,6.35 | 96.57,5.03 95.2,6.4 95.2,7.32 U7.14 | 106.12,6.35 106.17,6.4 106.17,10.46 108.2,12.5 110.64,12.5 111.25,13.11 114.5,13.11 U1.4 | 106.12,6.35 108.71,3.76 128.02,3.76 130.66,6.4 130.66,7.32 U8.14 | v59.54,9.04 59.38,8.89 | v84.94,4.98 v83.72,3.76 | v90.42,4.98 96.52,4.98 96.57,5.03
SPI_MOSI  (via drill 0.41)
  Top 0.203: v111.05,11.99 108.31,11.99 108.2,12.09 78.23,12.09 78.13,11.99 77.52,11.99 76.81,12.7 76.81,14.53 75.89,15.44 74.17,15.44 73.05,16.56 SERIAL.8
  Bottom 0.203: v111.05,11.99 111.15,11.89 114.5,11.89 U1.5
SPI_SCLK  (via drill 0.41)
  Top 0.203: v111.05,10.26 107.7,10.26 106.27,11.68 78.33,11.68 78.23,11.58 77.42,11.58 76.1,12.9 74.17,12.9 73.05,14.02 SERIAL.7
  Bottom 0.203: v111.05,10.26 111.96,9.35 114.5,9.35 U1.7

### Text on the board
_tsilk: SKAARHOJ 2013 | PCB-DISPARRAY4b | 1 | v10-13

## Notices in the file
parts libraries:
SparkFun: Licensing: CC v3.0 Share-Alike You are welcome to use this library for commercial purposes.
